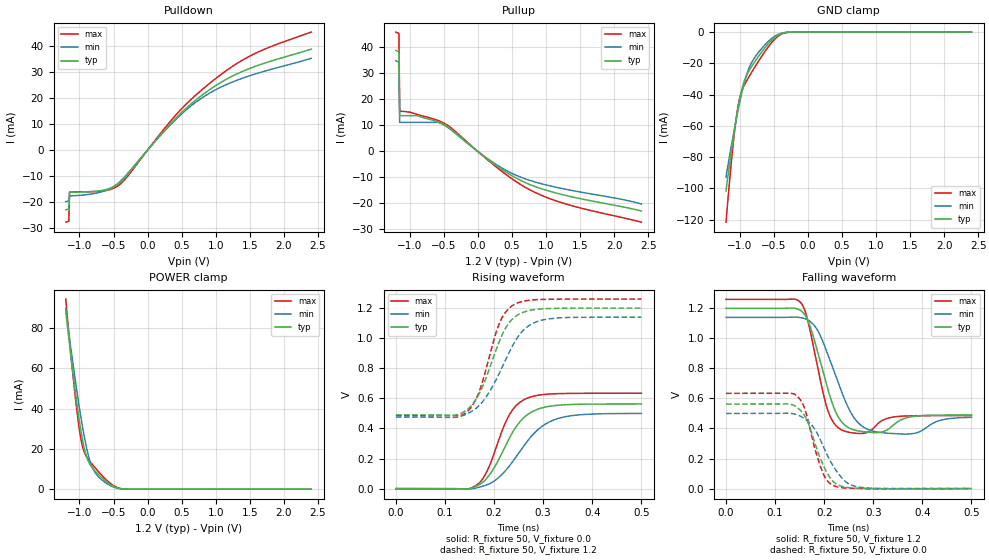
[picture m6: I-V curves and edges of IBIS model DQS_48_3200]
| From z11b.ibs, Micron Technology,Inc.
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| MODEL DQS_48_3200 (48 Ohm Data Strobe I/O with no ODT, 1600-3200Mbps)
[Model]   DQS_48_3200
Model_type   I/O
Vinl = 905.000mV
Vinh = 1015.000mV
Vmeas = 960.000mV
Vref = 1200.000mV
Cref = 0.0pF
Rref = 50.000Ohm
|   typ   min   max
|C_comp   0.780pF   0.730pF   0.830pF
C_comp_pullup   0.390pF   0.365pF   0.415pF
C_comp_pulldown   0.390pF   0.365pF   0.415pF
[Model Spec]
| Timing spec test load voltage corners
Vref   1.2000V   1.1400V   1.2600V
| Dynamic Overshoot Parameters from DDR4 Specification
|D_overshoot_ampl_h   0.40   NA   NA
|D_overshoot_ampl_l   0.40   NA   NA
|D_overshoot_area_h   0.0800n   NA   NA
|D_overshoot_area_l   0.0800n   NA   NA
[Voltage Range]   1.2000V   1.1400V   1.2600V
| Junction Temperature (Ambient temp is 35C typ, 95C min, 0C max)
[Temperature Range]   50.0   110.0   0.0
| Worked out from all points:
|   slope of the pulldown table from 0 to 0.18 V, typ, clamps not added: 32.4 ohm
|   slope of the pullup table from 0 to 0.18 V, typ, clamps not added: 49.2 ohm
|   GND clamp passes 1 mA (typ) near -0.39 V on its own axis
|   POWER clamp passes 1 mA (typ) near -0.48 V on its own axis
|   rising waveform, R_fixture 50, V_fixture 0.0: 20-80 % time 59ps typ, 74.4ps min, 47ps max; typ from 0 V to 0.563 V
|   rising waveform, R_fixture 50, V_fixture 1.2: 20-80 % time 52.1ps typ, 64.6ps min, 42.5ps max; typ from 0.49 V to 1.2 V
|   falling waveform, R_fixture 50, V_fixture 1.2: 20-80 % time 36.5ps typ, 46.3ps min, 30ps max; typ from 1.2 V to 0.49 V
|   falling waveform, R_fixture 50, V_fixture 0.0: 20-80 % time 38.9ps typ, 48.9ps min, 31.8ps max; typ from 0.563 V to 0 V
[Pulldown]
|   Voltage   I(typ)   I(min)   I(max)
-1.2V     -22.96mA   -19.84mA   -27.69mA
-1.156V   -22.64mA   -19.51mA   -27.34mA
-1.145V   -16.23mA   -17.61mA   -16.14mA
-687.3mV  -15.58mA   -16.14mA   -15.8mA
-534.5mV  -14.49mA   -14.58mA   -15.02mA
-414.5mV  -12.56mA   -12.33mA   -13.33mA
-294.5mV  -9.334mA   -9.047mA   -10.08mA
447.3mV   13.1mA     12.58mA    14.4mA
709.1mV   19.22mA    18.37mA    21.12mA
970.9mV   24.23mA    22.74mA    26.86mA
1.538V    31.71mA    28.84mA    36.56mA
2.4V      38.71mA    35.21mA    45.25mA
[GND_clamp]
|   Voltage   I(typ)   I(min)   I(max)
-1.2V     -101.7mA   -92.86mA   -121.7mA
-1.135V   -79.96mA   -75.85mA   -88.92mA
-1.08V    -63.49mA   -62.76mA   -65.41mA
-1.036V   -51.56mA   -52.84mA   -50.65mA
-992.7mV  -41.38mA   -43.58mA   -41.02mA
-927.3mV  -30.76mA   -31.6mA    -33.57mA
-872.7mV  -25.55mA   -24.13mA   -29.29mA
-818.2mV  -21.61mA   -19.01mA   -25.29mA
-621.8mV  -9.659mA   -7.799mA   -11.96mA
-436.4mV  -1.919mA   -1.478mA   -2.611mA
-229.1mV  -17.22uA   -19.75uA   -20.83uA
2.4V      0A         0A         0A
[Pullup]
|   Voltage   I(typ)   I(min)   I(max)
-1.2V     38.81mA    34.88mA    45.89mA
-1.156V   38.35mA    34.38mA    45.4mA
-1.145V   13.74mA    11.17mA    15.45mA
-883.6mV  13.71mA    11.17mA    14.18mA
-567.3mV  11.15mA    11.09mA    11.73mA
-392.7mV  8.512mA    8.301mA    9.088mA
0V        622.1nA    592.7nA    704.9nA
338.2mV   -6.633mA   -6.114mA   -7.357mA
600mV     -10.77mA   -9.589mA   -12.25mA
883.6mV   -13.91mA   -12.08mA   -16.31mA
1.385V    -17.5mA    -15.04mA   -20.91mA
2.4V      -22.93mA   -20.24mA   -27.22mA
[Power Clamp]
|   Voltage   I(typ)   I(min)   I(max)
-1.2V     88.83mA    89.6mA     94.34mA
-1.135V   68.72mA    72.21mA    70.04mA
-1.058V   47.72mA    53.58mA    44.98mA
-1.004V   34.46mA    41.14mA    30.26mA
-960mV    25.46mA    31.98mA    21.99mA
-894.5mV  16.03mA    20.41mA    16.05mA
-807.3mV  10.5mA     10.53mA    12.15mA
-709.1mV  6.909mA    5.768mA    8.277mA
-545.5mV  2.223mA    1.735mA    2.842mA
-436.4mV  532.8uA    427.3uA    716uA
-294.5mV  16.21uA    18.64uA    20.69uA
2.4V      0A         0A         0A
[Ramp]
|   typ   min   max
dV/dt_r   337.66m/58.99p   299.94m/74.37p   380.47m/47.05p
dV/dt_f   426.03m/36.45p   399.43m/46.27p   464.60m/29.97p
R_load = 50
[Rising Waveform]
R_fixture = 50
V_fixture = 0.0
|   Time   V(typ)   V(min)   V(max)
0s        2.779uV    7.506uV    1.603uV
144ps     -2.824mV   -2.947mV   -3.387mV
165ps     18.77mV    5.112mV    25.19mV
188ps     80.28mV    28.6mV     132.4mV
231ps     335.4mV    150mV      490mV
248ps     425.7mV    226.1mV    561.2mV
268ps     491.7mV    316.4mV    601.8mV
299ps     538.1mV    417.4mV    624.9mV
337ps     556mV      472.2mV    632mV
500ps     562.8mV    499.9mV    634.1mV
[Rising Waveform]
R_fixture   = 50
V_fixture   = 1.2
V_fixture_min = 1.14
V_fixture_max = 1.26
|   Time   V(typ)   V(min)   V(max)
0s        490mV      475.8mV    485.7mV
119ps     488.8mV    473.4mV    484.2mV
145ps     525.5mV    497.6mV    511mV
170ps     633.5mV    553.2mV    647.6mV
212ps     989.1mV    776.4mV    1.108V
225ps     1.076V     866.8mV    1.18V
242ps     1.14V      975.1mV    1.226V
266ps     1.179V     1.072V     1.249V
297ps     1.195V     1.12V      1.258V
500ps     1.2V       1.14V      1.26V
[Falling Waveform]
R_fixture   = 50
V_fixture   = 1.2
V_fixture_min = 1.14
V_fixture_max = 1.26
|   Time   V(typ)   V(min)   V(max)
0s        1.2V       1.14V      1.26V
152ps     1.185V     1.139V     1.239V
171ps     1.084V     1.114V     1.056V
206ps     677.9mV    905mV      534mV
236ps     442.4mV    639.8mV    389.7mV
267ps     385.2mV    445.5mV    367.5mV
305ps     372.6mV    378.5mV    418.5mV
376ps     477.3mV    364.1mV    484.3mV
437ps     489.3mV    454.8mV    485.6mV
500ps     489.9mV    474.3mV    485.7mV
[Falling Waveform]
R_fixture = 50
V_fixture = 0.0
|   Time   V(typ)   V(min)   V(max)
0s        562.8mV    500.2mV    634.1mV
144ps     542.8mV    492.4mV    618.2mV
161ps     480.2mV    462.9mV    524.9mV
180ps     310.4mV    399mV      277.9mV
197ps     163mV      289mV      106.4mV
207ps     96.79mV    217mV      49.25mV
221ps     38.82mV    136.2mV    16.84mV
245ps     8.249mV    42.28mV    3.127mV
272ps     1.745mV    9.108mV    397.8uV
500ps     7.18uV     -266.6uV   7.488uV
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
